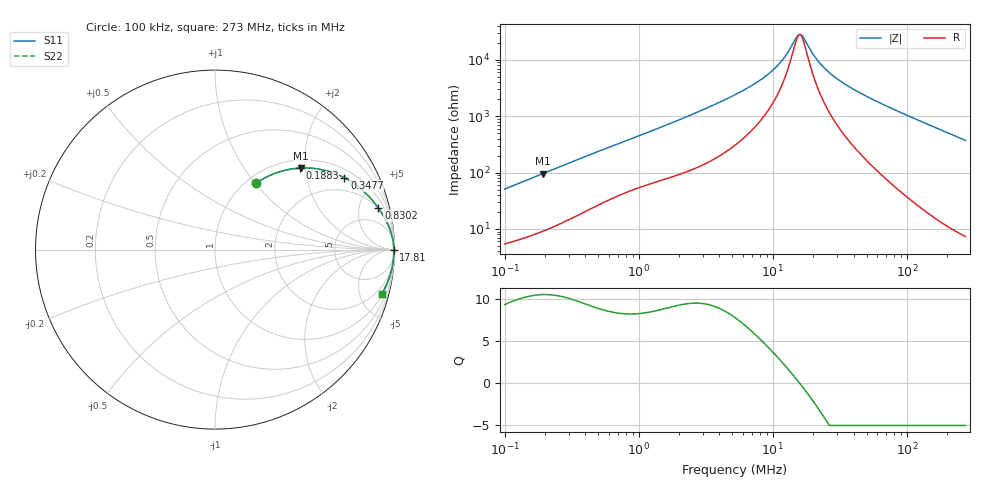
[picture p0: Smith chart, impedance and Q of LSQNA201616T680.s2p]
! LSQNA201616T680  S-PARAMETER MODEL  ( General Type )
! Model Generated by TAIYO YUDEN Corporation (http://www.ty-top.com)
! Version 2.0
! TAIYO YUDEN Control No. 100810NF25SB-FKC
! Copyright(c) 2007 TAIYO YUDEN CO.,LTD. All Rights Reserved.
! Product Description (link to TY-COMPAS)
! https://ds.yuden.co.jp/TYCOMPAS/or/detail?pn=LSQNA201616T680K&u=M
! Products Name : Inductors
! Characteristics :
!  Inductance : 68 uH , SRF(min) : 10 MHz , DC Resistance(max) : 3.9 Ohm
!  Rated Current : Saturation :90 mA , Temp Rise : 210 mA (40 degC)
!  Case Size : 2.0 x 1.6 / 0.079 x 0.063 [mm/inch] , Thickness : 1.6 / 0.063 [mm/inch]
!  (Conditions: Temperature = 25 degC , DC Bias Current/Voltage = 0A / 0V)
! External Node Assignments :
!  1  o---GGG---o  2
! GND o---------o GND
! Frequency Range : 0.1MHz  -  272.98108MHz  [ 402 STEP ]
# MHz S RI R 50
! Freq[MHz].  S11 Real  S11 Imag  S21 Real  S21 Imag  S12 Real  S12 Imag  S22 Real  S22 Imag
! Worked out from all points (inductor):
!   401 points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, 100 kHz to 273 MHz, reference 50 ohm
!   read as one part in series: L = 80 uH near 104 kHz
!   highest Q = 10.5 at 192.1 kHz (marker M1), where L = 78.9 uH
!   self-resonance near 15.82 MHz
!   S11 on the Smith chart (normalised r, x): 100 kHz: 1.11, +1.01; 188.3 kHz: 1.18, +1.87; 347.7 kHz: 1.34, +3.36; 830.2 kHz: 1.91, +7.50; 17.81 MHz: open; 273 MHz: 1.15, -7.45
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0.1  0.2294 0.3703  0.7706 -0.3703  0.7706 -0.3703  0.2294 0.3703
0.188317  0.4712 0.4539  0.5288 -0.4539  0.5288 -0.4539  0.4712 0.4539
0.192079  0.4799 0.4543  0.5201 -0.4543  0.5201 -0.4543  0.4799 0.4543
0.347689  0.7208 0.4003  0.2792 -0.4003  0.2792 -0.4003  0.7208 0.4003
0.376316  0.7466 0.3858  0.2534 -0.3858  0.2534 -0.3858  0.7466 0.3858
0.830167  0.91 0.2319  0.09 -0.2319  0.09 -0.2319  0.91 0.2319
1.416134  0.9579 0.1513  0.0421 -0.1513  0.0421 -0.1513  0.9579 0.1513
2.94406  0.9859 0.0765  0.0141 -0.0765  0.0141 -0.0765  0.9859 0.0765
5.329134  0.9932 0.0398  0.00681 -0.0398  0.00681 -0.0398  0.9932 0.0398
7.7602  0.9951 0.0237  0.00492 -0.0237  0.00492 -0.0237  0.9951 0.0237
10.23617  0.9959 0.0139  0.00414 -0.0139  0.00414 -0.0139  0.9959 0.0139
12.23068  0.9962 0.00811  0.00382 -0.00811  0.00382 -0.00811  0.9962 0.00811
15.50724  0.9964 0.000731  0.00355 -0.000731  0.00355 -0.000731  0.9964 0.000731
16.45529  0.9965 -0.0011  0.00351 0.0011  0.00351 0.0011  0.9965 -0.0011
17.81012  0.9965 -0.00355  0.00347 0.00355  0.00347 0.00355  0.9965 -0.00355
19.66158  0.9965 -0.00666  0.00345 0.00666  0.00345 0.00666  0.9965 -0.00666
23.96193  0.9965 -0.0131  0.0035 0.0131  0.0035 0.0131  0.9965 -0.0131
30.98818  0.9962 -0.0223  0.00376 0.0223  0.00376 0.0223  0.9962 -0.0223
44.24071  0.9954 -0.0377  0.00465 0.0377  0.00465 0.0377  0.9954 -0.0377
73.9896  0.9919 -0.0688  0.00805 0.0688  0.00805 0.0688  0.9919 -0.0688
144.9579  0.9769 -0.1375  0.0231 0.1375  0.0231 0.1375  0.9769 -0.1375
272.9811  0.9286 -0.2478  0.0714 0.2478  0.0714 0.2478  0.9286 -0.2478
